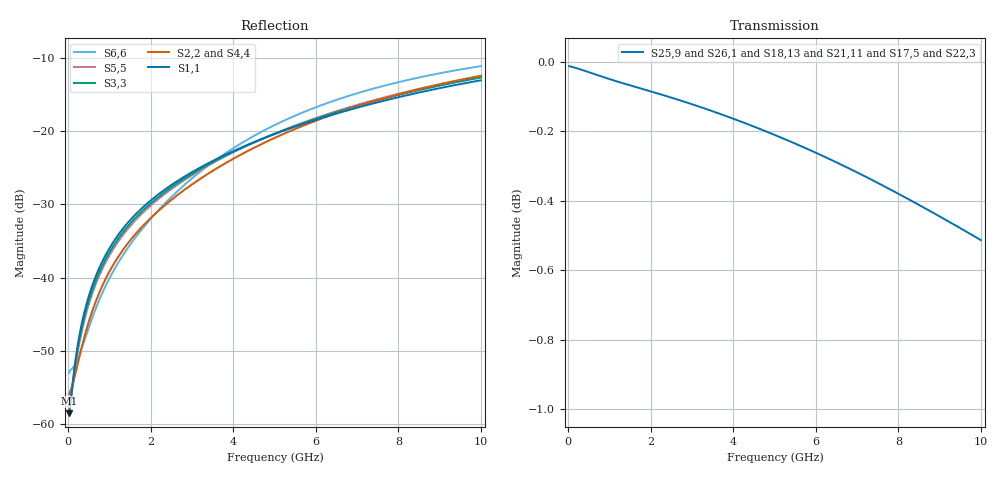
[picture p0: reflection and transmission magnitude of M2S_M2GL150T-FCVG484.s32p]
! M2S150T/M2GL150T FCVG484 S-parameter file
! Microsemi Corporation (c) 2020
!Initial ver: May 30, 2020
! Port::PIN_NAME::NET_NAME::S-parameter ports::PORTSIDE
! Port1:335:PCIE0_RXD_P_DIE::1::DIE
! Port2:337:PCIE0_RXD_N_DIE::2::DIE
! Port3:AA19:PCIE0_RXD_P_BGA::3::BGA
! Port4:AB19:PCIE0_RXD_N_BGA::4::BGA
! Port5:413:PCIE1_RXD_P_DIE::5::DIE
! Port6:415:PCIE1_RXD_N_DIE::6::DIE
! Port7:AB15:PCIE1_RXD_P_BGA::7::BGA
! Port8:AA15:PCIE1_RXD_N_BGA::8::BGA
! Port9:515:PCIE2_RXD_P_DIE::9::DIE
! Port10:517:PCIE2_RXD_N_DIE::10::DIE
! Port11:AB11:PCIE2_RXD_P_BGA::11::BGA
! Port12:AA11:PCIE2_RXD_N_BGA::12::BGA
! Port13:593:PCIE3_RXD_P_DIE::13::DIE
! Port14:595:PCIE3_RXD_N_DIE::14::DIE
! Port15:AB7:PCIE3_RXD_P_BGA::15::BGA
! Port16:AA7:PCIE3_RXD_N_BGA::16::BGA
! Port17:343:PCIE0_TXD_P_DIE::17::DIE
! Port18:341:PCIE0_TXD_N_DIE::18::DIE
! Port19:AB17:PCIE0_TXD_P_BGA::19::BGA
! Port20:AA17:PCIE0_TXD_N_BGA::20::BGA
! Port21:421:PCIE1_TXD_P_DIE::21::DIE
! Port22:419:PCIE1_TXD_N_DIE::22::DIE
! Port23:AA13:PCIE1_TXD_P_BGA::23::BGA
! Port24:AB13:PCIE1_TXD_N_BGA::24::BGA
! Port25:523:PCIE2_TXD_P_DIE::25::DIE
! Port26:521:PCIE2_TXD_N_DIE::26::DIE
! Port27:AA9:PCIE2_TXD_P_BGA::27::BGA
! Port28:AB9:PCIE2_TXD_N_BGA::28::BGA
! Port29:601:PCIE3_TXD_P_DIE::29::DIE
! Port30:599:PCIE3_TXD_N_DIE::30::DIE
! Port31:AA5:PCIE3_TXD_P_BGA::31::BGA
! Port32:AB5:PCIE3_TXD_N_BGA::32::BGA
!TouchstoneFormatFlag = 1
! GNDNET
! NETSLIST
! User Comments:
! Touchstone file exported from HFSS 3D Layout Design 2019.1.0
!  File:  D:/Ansys_EM_Models_2/M2S150T-FCVG484_SerDes_Analysis/658540AP0A.aedt
!  Generated:  8:33:08 PM  May 29, 2020
!  Design:  M2S150T-FCVG484_SerDes
!  Project:  658540AP0A
!  Setup:  HFSS Setup 1
!  Solution:  Sweep 1
! Terminal data exported
! Port[1] = PCIE2_RXD_N_BGA
! Port[2] = PCIE1_TXD_P_BGA
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# GHZ S MA R 50.000000
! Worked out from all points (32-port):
!   499 points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, 20.04 MHz to 10 GHz, reference 50 ohm
!   strongest paths, dB at 20.04 MHz, 2.505 GHz, 5.01 GHz, 7.515 GHz, 10 GHz:
!     S25,9: 0.0, -0.1, -0.2, -0.3, -0.5
!     S26,1: 0.0, -0.1, -0.2, -0.4, -0.5
!     S18,13: 0.0, -0.1, -0.2, -0.4, -0.5
!     S21,11: 0.0, -0.1, -0.2, -0.4, -0.6
!     S17,5: 0.0, -0.1, -0.2, -0.4, -0.6
!     S22,3: 0.0, -0.1, -0.2, -0.4, -0.6
!   lowest |S11| = -58.5 dB at 20.04 MHz (marker M1), VSWR 1.00, Z = 50.1 - j0.0236 ohm
!   |S11| at or under -10 dB: start of sweep to end of sweep
